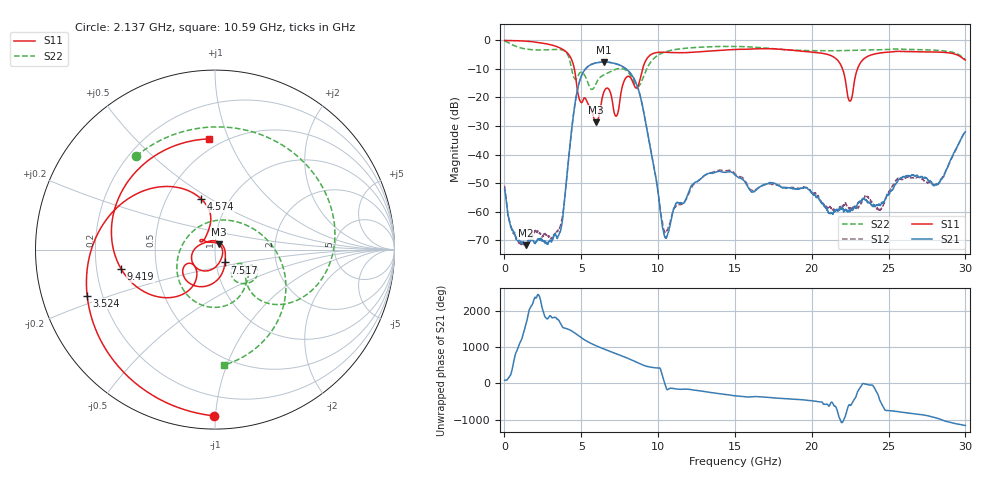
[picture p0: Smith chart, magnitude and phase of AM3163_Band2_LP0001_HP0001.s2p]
!Agilent Technologies,E8364B,MY43040894,A.07.50.67
!Agilent E8364B: A.07.50.67
!Date: Thursday, August 20, 2020 11:10:23
!Correction: S11(Full 2 Port(1,2))
!S21(Full 2 Port(1,2))
!S12(Full 2 Port(1,2))
!S22(Full 2 Port(1,2))
!S2P File: Measurements: S11, S21, S12, S22:
# Hz S  dB  R 50
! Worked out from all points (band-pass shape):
!   3201 points, 10 MHz to 30 GHz, reference 50 ohm
!   highest |S21| = -7.57 dB at 6.495 GHz (marker M1); lowest = -71.8 dB at 1.378 GHz (marker M2)
!   |S21| within 3 dB of the highest: 5.193 GHz to 8.042 GHz (2.849 GHz wide, 43.1 % of centre)
!   lowest |S11| = -28.7 dB at 5.971 GHz (marker M3), VSWR 1.08, Z = 52.1 + j3.08 ohm
!   |S11| at or under -10 dB: 4.55 GHz to 8.988 GHz (4.439 GHz wide, 65.6 % of centre); 22 GHz to 22.97 GHz (969.5 MHz wide, 4.31 % of centre)
!   |S22| runs from -17.2 to -0.3 dB; largest |S21 - S12| = 0.0034
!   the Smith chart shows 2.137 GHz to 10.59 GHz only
!   S11 on the Smith chart (normalised r, x): 2.137 GHz: 0.08, -0.99; 3.524 GHz: 0.14, -0.17; 4.574 GHz: 0.74, +0.46; 7.517 GHz: 1.10, -0.16; 9.419 GHz: 0.31, -0.09; 10.59 GHz: 0.43, +0.85
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1e7  -0.01 -2.6  -52.19 85.0  -50.97 30.2  -0.29 -12.0
5.629406e8  -0.08 -23.2  -66.97 157.9  -67.44 -80.2  -1.65 -87.9
1.378294e9  -0.26 -57.3  -71.81 163.4  -71.38 158.1  -3.00 -172.8
2.137416e9  -0.66 -90.2  -69.95 -99.7  -66.92 141.4  -3.34 130.0
3.524453e9  -2.42 -160.2  -68.33 -58.0  -66.18 82.9  -3.18 32.3
4.574103e9  -10.68 105.2  -22.76 -54.8  -22.78 -55.1  -13.45 -36.2
5.014581e9  -21.78 140.6  -12.36 169.7  -12.38 169.4  -11.19 -36.5
5.970512e9  -28.71 53.6  -7.87 -47.8  -7.88 -48.0  -14.99 -27.7
6.495338e9  -17.79 -112.7  -7.57 -139.3  -7.57 -139.4  -12.04 -44.4
7.516872e9  -20.86 -52.5  -8.67 55.3  -8.73 55.2  -9.84 -89.3
8.604009e9  -16.67 -138.9  -15.48 -140.3  -15.45 -140.1  -16.02 135.3
9.419362e9  -5.45 -168.3  -35.55 93.2  -35.47 92.9  -8.40 -11.7
1.000979e10  -4.19 138.5  -53.82 62.1  -53.53 57.8  -5.14 -55.3
1.059085e10  -4.18 93.2  -68.54 -176.0  -66.44 -157.0  -3.81 -85.4
1.217469e10  -4.19 -12.9  -50.88 -174.5  -51.64 -174.4  -2.57 -143.9
1.5005e10  -3.17 -144.2  -47.19 17.5  -46.76 17.4  -2.11 125.5
1.768536e10  -2.99 93.9  -50.45 -45.2  -50.75 -47.1  -3.00 27.3
2.000958e10  -4.10 -30.9  -53.44 -117.0  -53.28 -121.6  -3.61 -52.4
2.248376e10  -21.29 -104.1  -60.14 127.1  -59.00 169.9  -3.51 -121.3
2.500479e10  -4.10 -151.6  -54.01 -27.1  -53.06 -27.4  -3.19 177.4
2.818186e10  -4.09 109.7  -50.46 121.5  -50.38 120.2  -3.48 93.1
3e10  -6.89 42.2  -32.03 -76.8  -31.92 -76.6  -6.66 37.3
